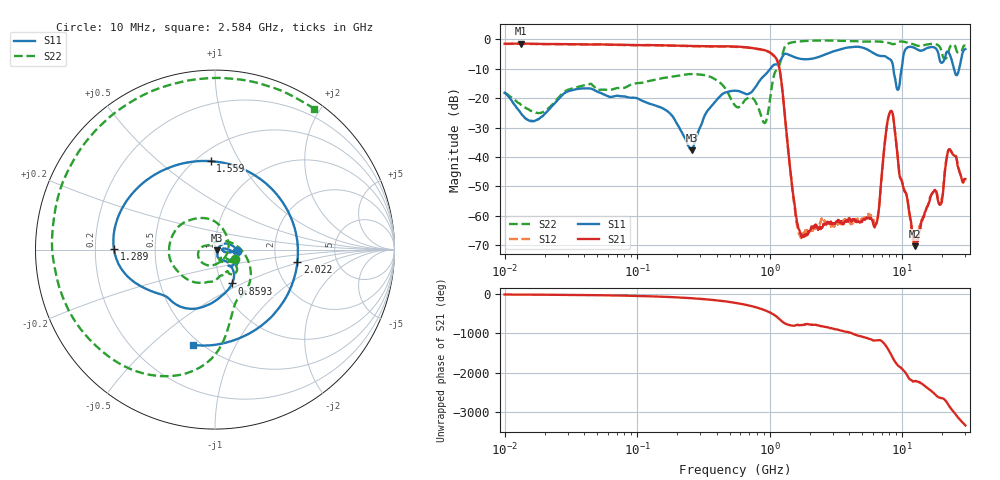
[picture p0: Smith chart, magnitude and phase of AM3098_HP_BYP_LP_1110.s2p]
!Agilent Technologies,E8364B,MY43040894,A.07.50.67
!Agilent E8364B: A.07.50.67
!Date: Wednesday, June 17, 2020 09:22:16
!Correction: S11(Full 2 Port(1,2))
!S21(Full 2 Port(1,2))
!S12(Full 2 Port(1,2))
!S22(Full 2 Port(1,2))
!S2P File: Measurements: S11, S21, S12, S22:Log Frequency Sweep
# Hz S  dB  R 50
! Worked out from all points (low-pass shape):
!   1601 points, 10 MHz to 30 GHz, reference 50 ohm
!   highest |S21| = -1.42 dB at 13.3 MHz (marker M1); lowest = -70.4 dB at 12.43 GHz (marker M2)
!   |S21| within 3 dB of the highest: start of sweep to 1.004 GHz
!   lowest |S11| = -37.7 dB at 257.3 MHz (marker M3), VSWR 1.03, Z = 51.3 - j0.349 ohm
!   |S11| at or under -10 dB: start of sweep to 1.012 GHz; 8.584 GHz to 9.91 GHz (1.326 GHz wide, 14.3 % of centre); 24.63 GHz to 26.93 GHz (2.298 GHz wide, 8.91 % of centre)
!   |S22| runs from -28.5 to -0.4 dB; largest |S21 - S12| = 0.015
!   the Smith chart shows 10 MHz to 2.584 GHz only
!   S11 on the Smith chart (normalised r, x): 10 MHz: 1.28, -0.01; 859.3 MHz: 1.12, -0.44; 1.289 GHz: 0.28, +0.00; 1.559 GHz: 0.59, +0.76; 2.022 GHz: 2.64, -0.45; 2.584 GHz: 0.45, -0.69
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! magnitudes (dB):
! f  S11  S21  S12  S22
! 10 MHz  -18.2  -1.5  -1.5  -18.1
! 13.3 MHz  -25.2  -1.4  -1.5  -22.3
! 38.04 MHz  -16.7  -1.7  -1.7  -15.8
! 144.7 MHz  -22.9  -2.0  -2.0  -13.4
! 257.3 MHz  -37.7  -2.2  -2.3  -11.8
! 547.7 MHz  -17.5  -2.5  -2.6  -22.5
! 859.3 MHz  -13.5  -3.4  -3.5  -25.8
! 1.137 GHz  -8.5  -7.0  -7.1  -10.3
! 1.289 GHz  -5.0  -23.7  -23.8  -3.0
! 1.559 GHz  -6.1  -57.5  -58.7  -0.8
! 2.022 GHz  -6.7  -64.8  -65.1  -0.4
! 2.084 GHz  -6.6  -63.9  -65.2  -0.4
! 2.584 GHz  -5.3  -63.1  -61.6  -0.4
! 6.296 GHz  -5.1  -63.2  -62.9  -0.7
! 7.926 GHz  -6.5  -25.9  -26.0  -1.2
! 9.256 GHz  -17.1  -40.2  -40.1  -1.1
! 12.43 GHz  -2.9  -70.4  -69.5  -1.8
! 17.04 GHz  -2.6  -52.1  -52.1  -1.5
! 19.61 GHz  -7.9  -56.0  -55.0  -3.4
! 22.67 GHz  -4.8  -37.3  -37.4  -3.3
! 25.82 GHz  -12.2  -40.9  -40.8  -4.0
! 30 GHz  -3.3  -47.5  -47.8  -2.1
